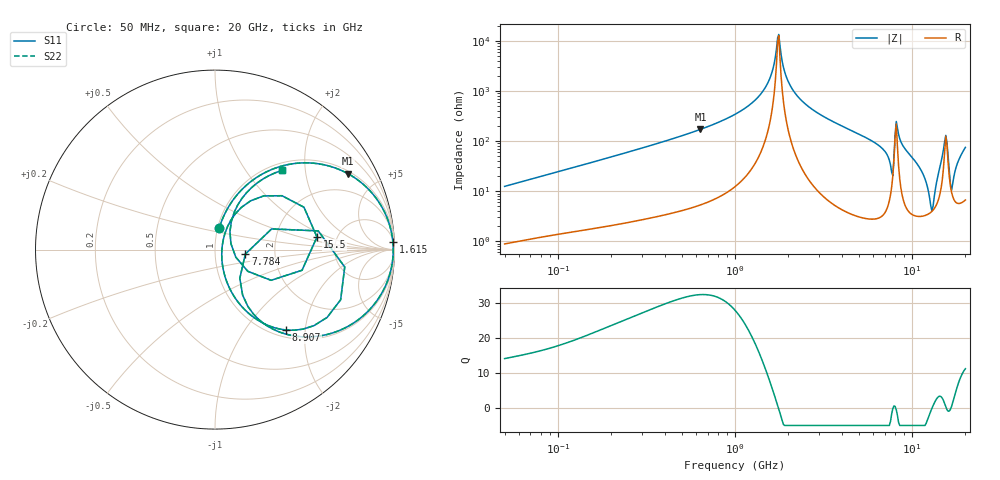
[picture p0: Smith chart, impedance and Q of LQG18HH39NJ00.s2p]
!Murata Part Number: LQG18HH39NJ00
!These Parameters are Measured in Series Mode Connection
!  o--[Z]--o
!Port1  Port2
!  o-------o
!Freq. Start=50[MHz] Stop=20[GHz], 401[Steps]
# Hz S RI R 50
!Freq.(Hz) S11(Real) S11(Imag) S21(Real) S21(Imag) S12(Real) S12(Imag) S22(Real) S22(Imag)
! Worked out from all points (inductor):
!   401 points, 50 MHz to 20 GHz, reference 50 ohm
!   read as one part in series: L = 39.4 nH near 51.52 MHz
!   highest Q = 32.4 at 638 MHz (marker M1), where L = 43 nH
!   self-resonance near 1.741 GHz
!   S11 on the Smith chart (normalised r, x): 50 MHz: 1.02, +0.25; 1.615 GHz: 9, +46; 7.784 GHz: 1.40, -0.07; 8.907 GHz: 1.14, -1.59; 15.5 GHz: 3.51, +0.73; 20 GHz: 1.13, +1.50
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5e7  0.0237 0.1208  0.9763 -0.1208  0.9763 -0.1208  0.0237 0.1208
1.364002e8  0.1108 0.29  0.8892 -0.29  0.8892 -0.29  0.1108 0.29
3.721004e8  0.4608 0.4816  0.5392 -0.4816  0.5392 -0.4816  0.4608 0.4816
6.380365e8  0.7417 0.4225  0.2583 -0.4225  0.2583 -0.4225  0.7417 0.4225
1e9  0.9142 0.2627  0.0858 -0.2627  0.0858 -0.2627  0.9142 0.2627
1.369645e9  0.9774 0.1202  0.0226 -0.1202  0.0226 -0.1202  0.9774 0.1202
1.614971e9  0.9911 0.0414  0.00887 -0.0414  0.00887 -0.0414  0.9911 0.0414
1.766834e9  0.9931 -0.00235  0.00692 0.00235  0.00692 0.00235  0.9931 -0.00235
2.05233e9  0.9874 -0.0759  0.0126 0.0759  0.0126 0.0759  0.9874 -0.0759
2.728004e9  0.9434 -0.2159  0.0566 0.2159  0.0566 0.2159  0.9434 -0.2159
5.944466e9  0.5036 -0.4864  0.4964 0.4864  0.4964 0.4864  0.5036 -0.4864
7.442007e9  0.1828 -0.3158  0.8172 0.3158  0.8172 0.3158  0.1828 -0.3158
7.784049e9  0.1689 -0.025  0.8311 0.025  0.8311 0.025  0.1689 -0.025
8.264682e9  0.7001 -0.2792  0.2999 0.2792  0.2999 0.2792  0.7001 -0.2792
8.907419e9  0.3971 -0.4482  0.6029 0.4482  0.6029 0.4482  0.3971 -0.4482
1.131968e10  0.0842 -0.2215  0.9158 0.2215  0.9158 0.2215  0.0842 -0.2215
1.295331e10  0.0383 -0.0023  0.9617 0.0023  0.9617 0.0023  0.0383 -0.0023
1.482269e10  0.271 0.2992  0.729 -0.2992  0.729 -0.2992  0.271 0.2992
1.550395e10  0.5681 0.0702  0.4319 -0.0702  0.4319 -0.0702  0.5681 0.0702
1.597544e10  0.3124 -0.1711  0.6876 0.1711  0.6876 0.1711  0.3124 -0.1711
1.670968e10  0.0885 0.0342  0.9115 -0.0342  0.9115 -0.0342  0.0885 0.0342
2e10  0.3724 0.4409  0.6276 -0.4409  0.6276 -0.4409  0.3724 0.4409
